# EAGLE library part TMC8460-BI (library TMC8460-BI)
ETHERCAT, IIC, PWM, RMII (EtherCAT), SPI, SSI ; BGA_VF400
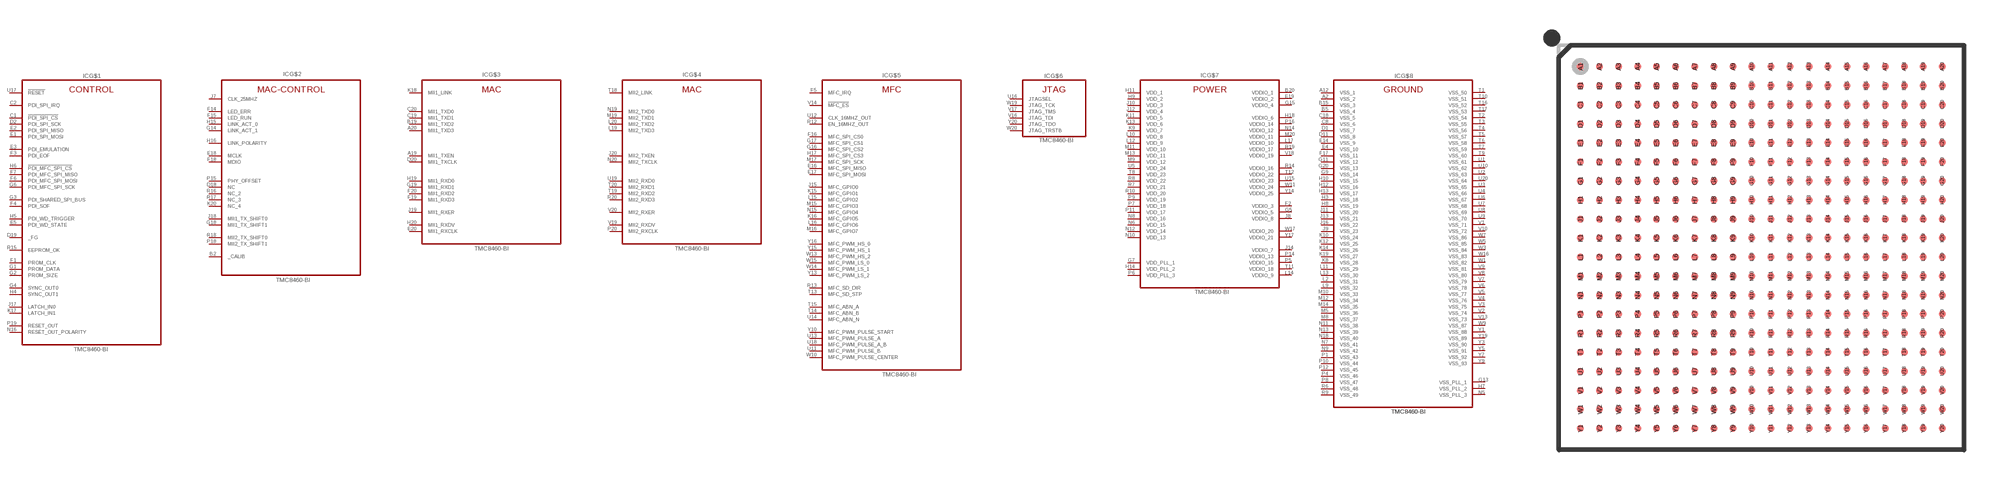
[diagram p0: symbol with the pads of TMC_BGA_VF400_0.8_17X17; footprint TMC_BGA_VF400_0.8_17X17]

Designator prefix IC; gates G$1=TMC8460_CONTROL G$2=TMC8460_MACCONTROL G$3=TMC8460_MAC G$4=TMC8460_MAC_2 G$5=TMC8460_MFC G$6=TMC8460_JTAG G$7=TMC8460_POWER G$8=TMC8460_GND

## TMC8460-BI (DESCRIPTION: ETHERCAT, IIC, PWM, RMII (EtherCAT), SPI, SSI ; BGA_VF400; GEOMETRY_HEIGHT: 1_51mm; MANUFACTURER: TRINAMIC; ORDERCODE-MANU1: TMC8460-BI; VALUE: TMC8460-BI)  [TMC_BGA_VF400_0.8_17X17]
A2  G$8:VSS_2  pas
A12  G$8:VSS_1  pas
A19  G$3:MII1_TXEN  pas
A20  G$3:MII1_TXD3  pas
B2  G$2:_CALIB  pas
B5  G$8:VSS_4  pas
B15  G$8:VSS_3  pas
B19  G$3:MII1_TXD2  pas
B20  G$7:VDDIO_1  pas
C1  G$1:!PDI_SPI_CS  pas
C2  G$1:PDI_SPI_IRQ  pas
C8  G$8:VSS_6  pas
C18  G$8:VSS_5  pas
C19  G$3:MII1_TXD1  pas
C20  G$3:MII1_TXD0  pas
D1  G$8:VSS_7  pas
D2  G$1:PDI_SPI_SCK  pas
D11  G$8:VSS_8  pas
D18  G$2:NC  pas
D19  G$1:_FG  pas
D20  G$3:MII1_TXCLK  pas
E1  G$1:PDI_SPI_MOSI  pas
E2  G$1:PDI_SPI_MISO  pas
E3  G$1:PDI_EMULATION  pas
E4  G$8:VSS_10  pas
E5  G$1:PDI_WD_STATE  pas
E14  G$8:VSS_9  pas
E16  G$5:MFC_SPI_MISO  pas
E17  G$5:MFC_SPI_MOSI  pas
E18  G$2:MCLK  pas
E19  G$7:VDDIO_2  pas
E20  G$3:MII1_RXCLK  pas
F1  G$1:PROM_CLK  pas
F2  G$7:VDDIO_3  pas
F3  G$1:PDI_EOF  pas
F4  G$1:PDI_SOF  pas
F5  G$5:MFC_IRQ  pas
F6  G$1:PDI_MFC_SPI_MOSI  pas
F7  G$1:PDI_MFC_SPI_MISO  pas
F14  G$2:LED_ERR  pas
F15  G$2:LED_RUN  pas
F16  G$5:MFC_SPI_CS0  pas
F17  G$8:VSS_11  pas
F18  G$2:MDIO  pas
F19  G$3:MII1_RXD3  pas
F20  G$3:MII1_RXD2  pas
G1  G$1:PROM_DATA  pas
G2  G$1:PROM_SIZE  pas
G3  G$1:PDI_SHARED_SPI_BUS  pas
G4  G$1:SYNC_OUT0  pas
G5  G$7:VDDIO_5  pas
G6  G$1:PDI_MFC_SPI_SCK  pas
G7  G$7:VDD_PLL_1  pas
G9  G$8:VSS_14  pas
G11  G$8:VSS_12  pas
G13  G$8:VSS_PLL_1  pas
G14  G$2:LINK_ACT_1  pas
G15  G$7:VDDIO_4  pas
G16  G$5:MFC_SPI_CS2  pas
G17  G$5:MFC_SPI_CS1  pas
G18  G$2:MII1_TX_SHIFT1  pas
G19  G$3:MII1_RXD1  pas
G20  G$8:VSS_13  pas
H3  G$8:VSS_18  pas
H4  G$1:SYNC_OUT1  pas
H5  G$1:PDI_WD_TRIGGER  pas
H6  G$1:!PDI_MFC_SPI_CS  pas
H7  G$8:VSS_PLL_2  pas
H8  G$8:VSS_19  pas
H9  G$7:VDD_2  pas
H10  G$8:VSS_15  pas
H11  G$7:VDD_1  pas
H12  G$8:VSS_16  pas
H13  G$8:VSS_17  pas
H14  G$7:VDD_PLL_2  pas
H15  G$2:LINK_ACT_0  pas
H16  G$2:LINK_POLARITY  pas
H17  G$5:MFC_SPI_CS3  pas
H18  G$7:VDDIO_6  pas
H19  G$3:MII1_RXD0  pas
H20  G$3:MII1_RXDV  pas
J7  G$2:CLK_25MHZ  pas
J8  G$7:VDDIO_8  pas
J9  G$8:VSS_23  pas
J10  G$7:VDD_3  pas
J11  G$8:VSS_20  pas
J12  G$7:VDD_4  pas
J13  G$8:VSS_21  pas
J14  G$7:VDDIO_7  pas
J15  G$5:MFC_GPIO0  pas
J16  G$8:VSS_22  pas
J17  G$1:LATCH_IN0  pas
J18  G$2:MII1_TX_SHIFT0  pas
J19  G$3:MII1_RXER  pas
J20  G$4:MII2_TXEN  pas
K8  G$8:VSS_28  pas
K9  G$7:VDD_7  pas
K10  G$8:VSS_24  pas
K11  G$7:VDD_5  pas
K12  G$8:VSS_25  pas
K13  G$7:VDD_6  pas
K14  G$8:VSS_26  pas
K15  G$5:MFC_GPIO1  pas
K16  G$5:MFC_GPIO5  pas
K17  G$1:LATCH_IN1  pas
K18  G$3:MII1_LINK  pas
K19  G$8:VSS_27  pas
K20  G$2:NC_4  pas
L2  G$8:VSS_31  pas
L9  G$8:VSS_32  pas
L10  G$7:VDD_8  pas
L11  G$8:VSS_29  pas
L12  G$7:VDD_9  pas
L13  G$8:VSS_30  pas
L14  G$7:VDDIO_9  pas
L15  G$5:MFC_GPIO2  pas
L16  G$5:MFC_GPIO6  pas
L17  G$7:VDDIO_10  pas
L19  G$4:MII2_TXD3  pas
L20  G$4:MII2_TXD2  pas
M5  G$8:VSS_36  pas
M8  G$8:VSS_37  pas
M9  G$7:VDD_12  pas
M10  G$8:VSS_33  pas
M11  G$7:VDD_10  pas
M12  G$8:VSS_34  pas
M13  G$7:VDD_11  pas
M14  G$8:VSS_35  pas
M15  G$5:MFC_GPIO3  pas
M16  G$5:MFC_GPIO7  pas
M17  G$5:MFC_SPI_SCK  pas
M19  G$4:MII2_TXD1  pas
M20  G$7:VDDIO_11  pas
N5  G$8:VSS_PLL_3  pas
N6  G$7:VDD_15  pas
N7  G$8:VSS_41  pas
N8  G$7:VDD_16  pas
N9  G$8:VSS_42  pas
N10  G$7:VDD_13  pas
N11  G$8:VSS_38  pas
N12  G$7:VDD_14  pas
N13  G$8:VSS_39  pas
N14  G$7:VDDIO_12  pas
N15  G$5:MFC_GPIO4  pas
N16  G$1:RESET_OUT_POLARITY  pas
N18  G$8:VSS_40  pas
N19  G$4:MII2_TXD0  pas
N20  G$4:MII2_TXCLK  pas
P1  G$8:VSS_43  pas
P4  G$8:VSS_46  pas
P5  G$7:VDDIO_15  pas
P6  G$7:VDD_PLL_3  pas
P7  G$7:VDD_18  pas
P8  G$8:VSS_47  pas
P9  G$7:VDD_19  pas
P10  G$8:VSS_44  pas
P11  G$7:VDD_17  pas
P12  G$8:VSS_45  pas
P14  G$7:VDDIO_13  pas
P15  G$2:PHY_OFFSET  pas
P16  G$7:VDDIO_14  pas
P18  G$2:MII2_TX_SHIFT1  pas
P19  G$1:RESET_OUT  pas
P20  G$4:MII2_RXCLK  pas
R6  G$8:VSS_48  pas
R7  G$7:VDD_21  pas
R8  G$7:VDD_22  pas
R9  G$8:VSS_49  pas
R10  G$7:VDD_20  pas
R12  G$5:EN_16MHZ_OUT  pas
R13  G$5:MFC_SD_DIR  pas
R14  G$7:VDDIO_16  pas
R15  G$1:EEPROM_OK  pas
R16  G$2:NC_2  pas
R17  G$2:NC_3  pas
R18  G$2:MII2_TX_SHIFT0  pas
R19  G$7:VDDIO_17  pas
R20  G$4:MII2_RXD3  pas
T1  G$8:VSS_50  pas
T2  G$8:VSS_54  pas
T3  G$8:VSS_55  pas
T4  G$8:VSS_56  pas
T5  G$8:VSS_57  pas
T6  G$8:VSS_58  pas
T7  G$8:VSS_59  pas
T8  G$7:VDD_23  pas
T9  G$8:VSS_60  pas
T10  G$8:VSS_51  pas
T11  G$7:VDDIO_18  pas
T12  G$7:VDDIO_22  pas
T13  G$5:MFC_SD_STP  pas
T14  G$5:MFC_ABN_B  pas
T15  G$5:MFC_ABN_A  pas
T16  G$8:VSS_52  pas
T17  G$8:VSS_53  pas
T18  G$4:MII2_LINK  pas
T19  G$4:MII2_RXD2  pas
T20  G$4:MII2_RXD1  pas
U1  G$8:VSS_61  pas
U2  G$8:VSS_63  pas
U3  G$8:VSS_65  pas
U4  G$8:VSS_66  pas
U5  G$7:VDD_24  pas
U6  G$8:VSS_67  pas
U7  G$8:VSS_68  pas
U8  G$8:VSS_69  pas
U9  G$8:VSS_70  pas
U10  G$8:VSS_62  pas
U11  G$5:MFC_PWM_PULSE_B  pas
U12  G$5:CLK_16MHZ_OUT  pas
U13  G$5:MFC_PWM_PULSE_A  pas
U14  G$5:MFC_ABN_N  pas
U15  G$7:VDDIO_23  pas
U16  G$6:JTAGSEL  pas
U17  G$1:!RESET!  pas
U18  G$5:MFC_PWM_PULSE_A_B  pas
U19  G$4:MII2_RXD0  pas
U20  G$8:VSS_64  pas
V1  G$8:VSS_71  pas
V2  G$8:VSS_74  pas
V3  G$8:VSS_75  pas
V4  G$8:VSS_76  pas
V5  G$8:VSS_77  pas
V6  G$8:VSS_78  pas
V7  G$8:VSS_79  pas
V8  G$8:VSS_80  pas
V9  G$8:VSS_81  pas
V10  G$8:VSS_72  pas
V13  G$8:VSS_73  pas
V14  G$5:!MFC_ES  pas
V16  G$6:JTAG_TDI  pas
V17  G$6:JTAG_TMS  pas
V18  G$7:VDDIO_19  pas
V19  G$4:MII2_RXDV  pas
V20  G$4:MII2_RXER  pas
W1  G$8:VSS_82  pas
W3  G$8:VSS_84  pas
W5  G$8:VSS_85  pas
W7  G$8:VSS_86  pas
W9  G$8:VSS_87  pas
W10  G$5:MFC_PWM_PULSE_CENTER  pas
W11  G$7:VDDIO_24  pas
W13  G$5:MFC_PWM_HS_2  pas
W14  G$5:MFC_PWM_LS_1  pas
W15  G$5:MFC_PWM_LS_0  pas
W16  G$8:VSS_83  pas
W17  G$7:VDDIO_20  pas
W19  G$6:JTAG_TCK  pas
W20  G$6:JTAG_TRSTB  pas
Y1  G$8:VSS_88  pas
Y3  G$8:VSS_90  pas
Y5  G$8:VSS_91  pas
Y7  G$8:VSS_92  pas
Y9  G$8:VSS_93  pas
Y10  G$5:MFC_PWM_PULSE_START  pas
Y13  G$5:MFC_PWM_LS_2  pas
Y14  G$7:VDDIO_25  pas
Y15  G$5:MFC_PWM_HS_1  pas
Y16  G$5:MFC_PWM_HS_0  pas
Y17  G$7:VDDIO_21  pas
Y19  G$8:VSS_89  pas
Y20  G$6:JTAG_TDO  pas

## Footprint TMC_BGA_VF400_0.8_17X17 (pad centres in mm)
smd 0.3 x 0.3: A1 -7.6,7.6; A2 -6.8,7.6; A3 -6,7.6; A4 -5.2,7.6; A5 -4.4,7.6; A6 -3.6,7.6; A7 -2.8,7.6; A8 -2,7.6; A9 -1.2,7.6; A10 -0.4,7.6; A11 0.4,7.6; A12 1.2,7.6; A13 2,7.6; A14 2.8,7.6; A15 3.6,7.6; A16 4.4,7.6; A17 5.2,7.6; A18 6,7.6; A19 6.8,7.6; A20 7.6,7.6; B1 -7.6,6.8; B2 -6.8,6.8; B3 -6,6.8; B4 -5.2,6.8; B5 -4.4,6.8; B6 -3.6,6.8; B7 -2.8,6.8; B8 -2,6.8; B9 -1.2,6.8; B10 -0.4,6.8; B11 0.4,6.8; B12 1.2,6.8; B13 2,6.8; B14 2.8,6.8; B15 3.6,6.8; B16 4.4,6.8; B17 5.2,6.8; B18 6,6.8; B19 6.8,6.8; B20 7.6,6.8; C1 -7.6,6; C2 -6.8,6; C3 -6,6; C4 -5.2,6; C5 -4.4,6; C6 -3.6,6; C7 -2.8,6; C8 -2,6; C9 -1.2,6; C10 -0.4,6; C11 0.4,6; C12 1.2,6; C13 2,6; C14 2.8,6; C15 3.6,6; C16 4.4,6; C17 5.2,6; C18 6,6; C19 6.8,6; C20 7.6,6; D1 -7.6,5.2; D2 -6.8,5.2; D3 -6,5.2; D4 -5.2,5.2; D5 -4.4,5.2; D6 -3.6,5.2; D7 -2.8,5.2; D8 -2,5.2; D9 -1.2,5.2; D10 -0.4,5.2; D11 0.4,5.2; D12 1.2,5.2; D13 2,5.2; D14 2.8,5.2; D15 3.6,5.2; D16 4.4,5.2; D17 5.2,5.2; D18 6,5.2; D19 6.8,5.2; D20 7.6,5.2; E1 -7.6,4.4; E2 -6.8,4.4; E3 -6,4.4; E4 -5.2,4.4; E5 -4.4,4.4; E6 -3.6,4.4; E7 -2.8,4.4; E8 -2,4.4; E9 -1.2,4.4; E10 -0.4,4.4; E11 0.4,4.4; E12 1.2,4.4; E13 2,4.4; E14 2.8,4.4; E15 3.6,4.4; E16 4.4,4.4; E17 5.2,4.4; E18 6,4.4; E19 6.8,4.4; E20 7.6,4.4; F1 -7.6,3.6; F2 -6.8,3.6; F3 -6,3.6; F4 -5.2,3.6; F5 -4.4,3.6; F6 -3.6,3.6; F7 -2.8,3.6; F8 -2,3.6; F9 -1.2,3.6; F10 -0.4,3.6; F11 0.4,3.6; F12 1.2,3.6; F13 2,3.6; F14 2.8,3.6; F15 3.6,3.6; F16 4.4,3.6; F17 5.2,3.6; F18 6,3.6; F19 6.8,3.6; F20 7.6,3.6; G1 -7.6,2.8; G2 -6.8,2.8; G3 -6,2.8; G4 -5.2,2.8; G5 -4.4,2.8; G6 -3.6,2.8; G7 -2.8,2.8; G8 -2,2.8; G9 -1.2,2.8; G10 -0.4,2.8; G11 0.4,2.8; G12 1.2,2.8; G13 2,2.8; G14 2.8,2.8; G15 3.6,2.8; G16 4.4,2.8; G17 5.2,2.8; G18 6,2.8; G19 6.8,2.8; G20 7.6,2.8; H1 -7.6,2; H2 -6.8,2; H3 -6,2; H4 -5.2,2; H5 -4.4,2; H6 -3.6,2; H7 -2.8,2; H8 -2,2; H9 -1.2,2; H10 -0.4,2; H11 0.4,2; H12 1.2,2; H13 2,2; H14 2.8,2; H15 3.6,2; H16 4.4,2; H17 5.2,2; H18 6,2; H19 6.8,2; H20 7.6,2; J1 -7.6,1.2; J2 -6.8,1.2; J3 -6,1.2; J4 -5.2,1.2; J5 -4.4,1.2; J6 -3.6,1.2; J7 -2.8,1.2; J8 -2,1.2; J9 -1.2,1.2; J10 -0.4,1.2; J11 0.4,1.2; J12 1.2,1.2; J13 2,1.2; J14 2.8,1.2; J15 3.6,1.2; J16 4.4,1.2; J17 5.2,1.2; J18 6,1.2; J19 6.8,1.2; J20 7.6,1.2; K1 -7.6,0.4; K2 -6.8,0.4; K3 -6,0.4; K4 -5.2,0.4; K5 -4.4,0.4; K6 -3.6,0.4; K7 -2.8,0.4; K8 -2,0.4; K9 -1.2,0.4; K10 -0.4,0.4; K11 0.4,0.4; K12 1.2,0.4; K13 2,0.4; K14 2.8,0.4; K15 3.6,0.4; K16 4.4,0.4; K17 5.2,0.4; K18 6,0.4; K19 6.8,0.4; K20 7.6,0.4; L1 -7.6,-0.4; L2 -6.8,-0.4; L3 -6,-0.4; L4 -5.2,-0.4; L5 -4.4,-0.4; L6 -3.6,-0.4; L7 -2.8,-0.4; L8 -2,-0.4; L9 -1.2,-0.4; L10 -0.4,-0.4; L11 0.4,-0.4; L12 1.2,-0.4; L13 2,-0.4; L14 2.8,-0.4; L15 3.6,-0.4; L16 4.4,-0.4; L17 5.2,-0.4; L18 6,-0.4; L19 6.8,-0.4; L20 7.6,-0.4; M1 -7.6,-1.2; M2 -6.8,-1.2; M3 -6,-1.2; M4 -5.2,-1.2; M5 -4.4,-1.2; M6 -3.6,-1.2; M7 -2.8,-1.2; M8 -2,-1.2; M9 -1.2,-1.2; M10 -0.4,-1.2; M11 0.4,-1.2; M12 1.2,-1.2; M13 2,-1.2; M14 2.8,-1.2; M15 3.6,-1.2; M16 4.4,-1.2; M17 5.2,-1.2; M18 6,-1.2; M19 6.8,-1.2; M20 7.6,-1.2; N1 -7.6,-2; N2 -6.8,-2; N3 -6,-2; N4 -5.2,-2; N5 -4.4,-2; N6 -3.6,-2; N7 -2.8,-2; N8 -2,-2; N9 -1.2,-2; N10 -0.4,-2; N11 0.4,-2; N12 1.2,-2; N13 2,-2; N14 2.8,-2; N15 3.6,-2; N16 4.4,-2; N17 5.2,-2; N18 6,-2; N19 6.8,-2; N20 7.6,-2; P1 -7.6,-2.8; P2 -6.8,-2.8; P3 -6,-2.8; P4 -5.2,-2.8; P5 -4.4,-2.8; P6 -3.6,-2.8; P7 -2.8,-2.8; P8 -2,-2.8; P9 -1.2,-2.8; P10 -0.4,-2.8; P11 0.4,-2.8; P12 1.2,-2.8; P13 2,-2.8; P14 2.8,-2.8; P15 3.6,-2.8; P16 4.4,-2.8; P17 5.2,-2.8; P18 6,-2.8; P19 6.8,-2.8; P20 7.6,-2.8; R1 -7.6,-3.6; R2 -6.8,-3.6; R3 -6,-3.6; R4 -5.2,-3.6; R5 -4.4,-3.6; R6 -3.6,-3.6; R7 -2.8,-3.6; R8 -2,-3.6; R9 -1.2,-3.6; R10 -0.4,-3.6; R11 0.4,-3.6; R12 1.2,-3.6; R13 2,-3.6; R14 2.8,-3.6; R15 3.6,-3.6; R16 4.4,-3.6; R17 5.2,-3.6; R18 6,-3.6; R19 6.8,-3.6; R20 7.6,-3.6; T1 -7.6,-4.4; T2 -6.8,-4.4; T3 -6,-4.4; T4 -5.2,-4.4; T5 -4.4,-4.4; T6 -3.6,-4.4; T7 -2.8,-4.4; T8 -2,-4.4; T9 -1.2,-4.4; T10 -0.4,-4.4; T11 0.4,-4.4; T12 1.2,-4.4; T13 2,-4.4; T14 2.8,-4.4; T15 3.6,-4.4; T16 4.4,-4.4; T17 5.2,-4.4; T18 6,-4.4; T19 6.8,-4.4; T20 7.6,-4.4; U1 -7.6,-5.2; U2 -6.8,-5.2; U3 -6,-5.2; U4 -5.2,-5.2; U5 -4.4,-5.2; U6 -3.6,-5.2; U7 -2.8,-5.2; U8 -2,-5.2; U9 -1.2,-5.2; U10 -0.4,-5.2; U11 0.4,-5.2; U12 1.2,-5.2; U13 2,-5.2; U14 2.8,-5.2; U15 3.6,-5.2; U16 4.4,-5.2; U17 5.2,-5.2; U18 6,-5.2; U19 6.8,-5.2; U20 7.6,-5.2; V1 -7.6,-6; V2 -6.8,-6; V3 -6,-6; V4 -5.2,-6; V5 -4.4,-6; V6 -3.6,-6; V7 -2.8,-6; V8 -2,-6; V9 -1.2,-6; V10 -0.4,-6; V11 0.4,-6; V12 1.2,-6; V13 2,-6; V14 2.8,-6; V15 3.6,-6; V16 4.4,-6; V17 5.2,-6; V18 6,-6; V19 6.8,-6; V20 7.6,-6; W1 -7.6,-6.8; W2 -6.8,-6.8; W3 -6,-6.8; W4 -5.2,-6.8; W5 -4.4,-6.8; W6 -3.6,-6.8; W7 -2.8,-6.8; W8 -2,-6.8; W9 -1.2,-6.8; W10 -0.4,-6.8; W11 0.4,-6.8; W12 1.2,-6.8; W13 2,-6.8; W14 2.8,-6.8; W15 3.6,-6.8; W16 4.4,-6.8; W17 5.2,-6.8; W18 6,-6.8; W19 6.8,-6.8; W20 7.6,-6.8; Y1 -7.6,-7.6; Y2 -6.8,-7.6; Y3 -6,-7.6; Y4 -5.2,-7.6; Y5 -4.4,-7.6; Y6 -3.6,-7.6; Y7 -2.8,-7.6; Y8 -2,-7.6; Y9 -1.2,-7.6; Y10 -0.4,-7.6; Y11 0.4,-7.6; Y12 1.2,-7.6; Y13 2,-7.6; Y14 2.8,-7.6; Y15 3.6,-7.6; Y16 4.4,-7.6; Y17 5.2,-7.6; Y18 6,-7.6; Y19 6.8,-7.6; Y20 7.6,-7.6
